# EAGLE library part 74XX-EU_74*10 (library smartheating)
Triple 3-input NAND gate
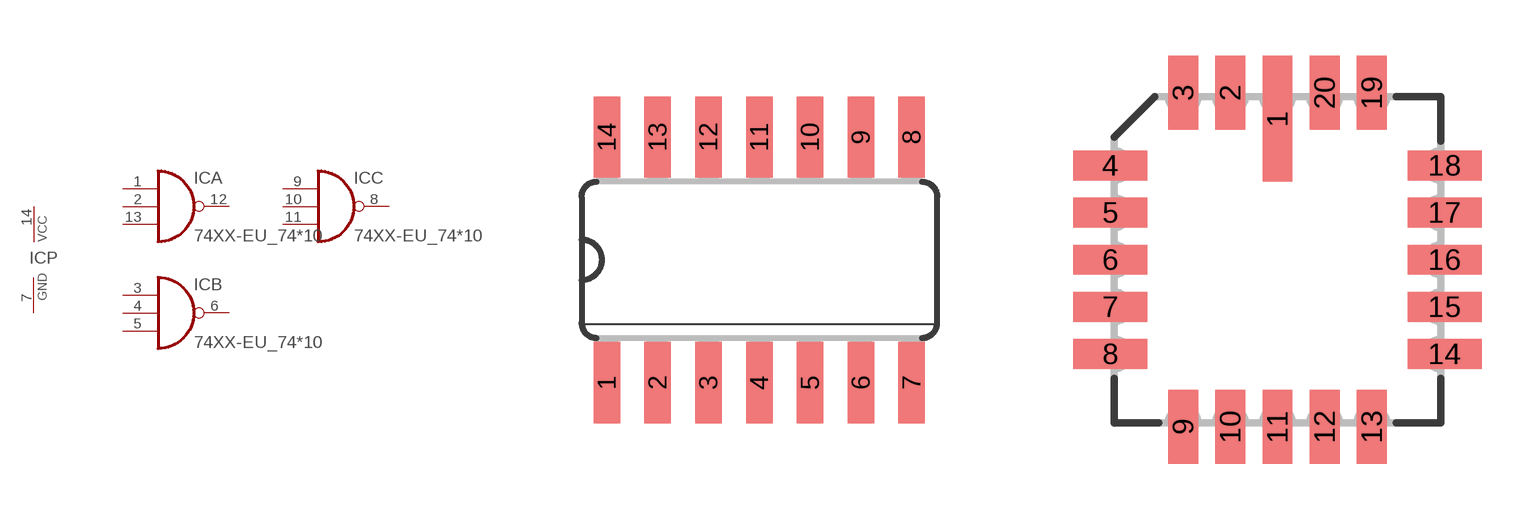
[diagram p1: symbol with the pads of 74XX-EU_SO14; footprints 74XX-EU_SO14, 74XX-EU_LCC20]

Designator prefix IC; gates A=74XX-EU_7410 B=74XX-EU_7410 C=74XX-EU_7410 P=74XX-EU_PWRN

## 74XX-EU_7410D, 74XX-EU_74AC10D, 74XX-EU_74ACT10D, 74XX-EU_74ALS10D, 74XX-EU_74AS10D, 74XX-EU_74HC10D, 74XX-EU_74HCT10D, 74XX-EU_74LS10D, 74XX-EU_74S10D  [74XX-EU_SO14]
1  A:I0  in
2  A:I1  in
3  B:I0  in
4  B:I1  in
5  B:I2  in
6  B:O  out
7  P:GND  pwr
8  C:O  out
9  C:I0  in
10  C:I1  in
11  C:I2  in
12  A:O  out
13  A:I2  in
14  P:VCC  pwr

## 74XX-EU_7410FK, 74XX-EU_74AC10FK, 74XX-EU_74ACT10FK, 74XX-EU_74ALS10FK, 74XX-EU_74AS10FK, 74XX-EU_74HC10FK, 74XX-EU_74HCT10FK, 74XX-EU_74LS10FK, 74XX-EU_74S10FK  [74XX-EU_LCC20]
2  A:I0  in
3  A:I1  in
4  B:I0  in
6  B:I1  in
8  B:I2  in
9  B:O  out
10  P:GND  pwr
12  C:O  out
13  C:I0  in
14  C:I1  in
16  C:I2  in
18  A:O  out
19  A:I2  in
20  P:VCC  pwr

## 74XX-EU_7410N, 74XX-EU_74AC10N, 74XX-EU_74ACT10N, 74XX-EU_74ALS10N, 74XX-EU_74AS10N, 74XX-EU_74HC10N, 74XX-EU_74HCT10N, 74XX-EU_74LS10N, 74XX-EU_74S10N  [74XX-EU_DIL14]
Pads as for 74XX-EU_SO14

## Footprint 74XX-EU_SO14 (pad centres in mm)
Small Outline package 150 mil
smd 0.66 x 2.032: 1 -3.81,-3.073; 2 -2.54,-3.073; 3 -1.27,-3.073; 4 0,-3.073; 5 1.27,-3.073; 6 2.54,-3.073; 7 3.81,-3.073; 8 3.81,3.073; 9 2.54,3.073; 10 1.27,3.073; 11 0,3.073; 12 -1.27,3.073; 13 -2.54,3.073; 14 -3.81,3.073

## Footprint 74XX-EU_LCC20 (pad centres in mm)
Leadless Chip Carrier Ceramic Package
smd 0.8 x 3.4: 1 0,3.8
smd 0.8 x 2: 2 -1.27,4.5; 3 -2.54,4.5; 9 -2.54,-4.5; 10 -1.27,-4.5; 11 0,-4.5; 12 1.27,-4.5; 13 2.54,-4.5; 19 2.54,4.5; 20 1.27,4.5
smd 2 x 0.8: 4 -4.5,2.54; 5 -4.5,1.27; 6 -4.5,0; 7 -4.5,-1.27; 8 -4.5,-2.54; 14 4.5,-2.54; 15 4.5,-1.27; 16 4.5,0; 17 4.5,1.27; 18 4.5,2.54

## Footprint 74XX-EU_DIL14 (pad centres in mm)
Dual In Line Package
drill 0.813 long: 1 -7.62,-3.81; 2 -5.08,-3.81; 3 -2.54,-3.81; 4 0,-3.81; 5 2.54,-3.81; 6 5.08,-3.81; 7 7.62,-3.81; 8 7.62,3.81; 9 5.08,3.81; 10 2.54,3.81; 11 0,3.81; 12 -2.54,3.81; 13 -5.08,3.81; 14 -7.62,3.81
